INTERFACE I_Cylinder

PROPERTY bState_AtBasePos : BOOL
GET
END_GET
END_PROPERTY

PROPERTY bState_AtWorkPos : BOOL
GET
END_GET
END_PROPERTY

PROPERTY bState_MoveToWork : BOOL
GET
END_GET
END_PROPERTY

METHOD MoveToBase
VAR_INPUT
END_VAR
END_METHOD

METHOD MoveToWork
VAR_INPUT
END_VAR
END_METHOD

METHOD Reset
VAR_INPUT
END_VAR
END_METHOD

END_INTERFACE
